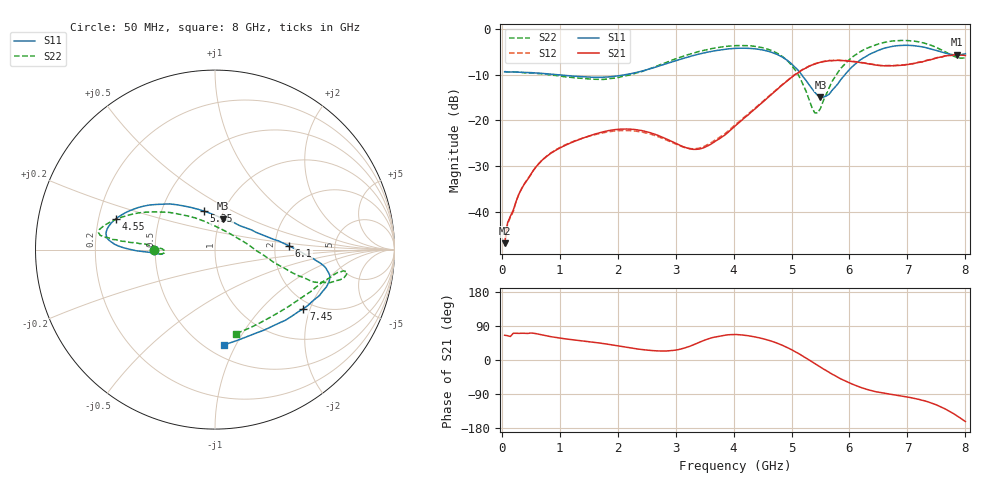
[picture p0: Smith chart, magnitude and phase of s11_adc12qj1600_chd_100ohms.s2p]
#  HZ  S  DB  R  100.00
! Rohde & Schwarz ZVA24 4Ports - Version 4.10 - 1145.1110k26 SN: 100644
! Date: 2020-07-21 15:53:25
! Measurements: S11 S31 S13 S33
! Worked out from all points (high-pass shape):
!   160 points, 50 MHz to 8 GHz, reference 100 ohm
!   highest |S21| = -5.67 dB at 7.85 GHz (marker M1); lowest = -46.9 dB at 50 MHz (marker M2)
!   |S21| within 3 dB of the highest: 5.236 GHz to end of sweep
!   lowest |S11| = -15.0 dB at 5.5 GHz (marker M3), VSWR 1.43, Z = 103 + j36.7 ohm
!   |S11| at or under -10 dB: 921 MHz to 2.149 GHz (1.228 GHz wide, 80 % of centre); 5.172 GHz to 5.924 GHz (752.2 MHz wide, 13.6 % of centre)
!   |S22| runs from -18.4 to -2.6 dB; largest |S21 - S12| = 0.0041
!   S11 on the Smith chart (normalised r, x): 50 MHz: 0.49, -0.00; 4.55 GHz: 0.27, +0.14; 5.35 GHz: 0.81, +0.37; 6.1 GHz: 2.39, +0.13; 7.45 GHz: 1.77, -1.80; 8 GHz: 0.60, -0.89
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5e7  -9.40 -179.3  -46.88 65.3  -47.53 64.6  -9.35 -179.6
1e8  -9.44 -179.8  -42.50 64.1  -42.69 65.1  -9.43 -179.7
2.5e8  -9.47 -178.6  -37.71 70.4  -37.64 71.4  -9.43 -178.5
5.5e8  -9.62 -177.2  -30.90 70.6  -30.89 70.6  -9.72 -176.9
8.5e8  -9.91 -176.1  -27.21 61.5  -27.12 61.6  -10.11 -175.5
1.4e9  -10.50 -175.2  -23.91 50.2  -23.89 48.7  -10.84 -176.1
2.05e9  -10.21 -175.8  -21.94 36.2  -22.26 35.8  -10.52 178.9
2.7e9  -8.19 -178.1  -23.32 23.9  -23.59 25.5  -8.02 175.3
3.4e9  -5.54 178.3  -26.32 46.0  -26.12 48.7  -4.97 174.4
4.05e9  -4.27 172.4  -21.00 67.2  -20.78 67.0  -3.68 171.8
4.55e9  -4.76 162.8  -15.51 54.5  -15.38 54.2  -4.31 165.7
5e9  -7.66 142.6  -10.64 27.3  -10.56 27.0  -7.95 148.4
5.35e9  -13.04 105.7  -7.94 -4.4  -7.89 -4.7  -17.12 96.2
5.4e9  -13.86 97.0  -7.71 -9.2  -7.64 -9.4  -18.38 75.3
5.5e9  -14.97 75.4  -7.31 -18.8  -7.26 -19.1  -17.40 31.1
5.75e9  -12.77 28.7  -6.93 -41.2  -6.87 -41.5  -10.52 -9.1
6.1e9  -7.72 3.1  -7.20 -66.7  -7.16 -66.9  -5.73 -17.5
6.7e9  -3.96 -10.3  -8.08 -90.2  -8.03 -90.3  -2.74 -12.8
7.1e9  -3.67 -18.4  -7.64 -100.7  -7.59 -100.9  -2.68 -9.5
7.45e9  -4.54 -33.8  -6.59 -115.5  -6.53 -115.8  -3.81 -14.9
7.85e9  -5.74 -68.7  -5.67 -146.8  -5.63 -147.0  -6.24 -50.5
8e9  -5.46 -84.8  -5.84 -162.3  -5.79 -162.6  -6.33 -75.7
